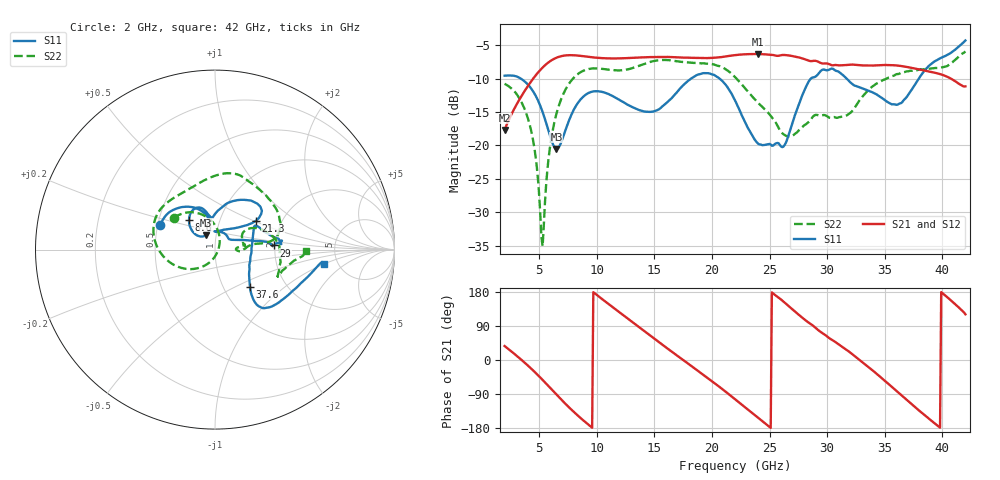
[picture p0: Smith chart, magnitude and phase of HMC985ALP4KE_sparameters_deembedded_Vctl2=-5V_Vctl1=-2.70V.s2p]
!s2p File: Measurements: S11, S21, S12, S22
# GHz S dB R 50.0
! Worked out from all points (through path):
!   401 points, 2 GHz to 42 GHz, reference 50 ohm
!   highest |S21| = -6.29 dB at 24 GHz (marker M1); lowest = -17.7 dB at 2 GHz (marker M2)
!   lowest |S11| = -20.5 dB at 6.5 GHz (marker M3), VSWR 1.21, Z = 44.8 + j7.26 ohm
!   |S11| at or under -10 dB: 3.42 GHz to 18.17 GHz (14.76 GHz wide, 137 % of centre); 20.67 GHz to 28.58 GHz (7.911 GHz wide, 32.1 % of centre); 31.7 GHz to 37.95 GHz (6.251 GHz wide, 18 % of centre)
!   |S22| runs from -35.1 to -5.9 dB; largest |S21 - S12| = 0.00063
!   S11 on the Smith chart (normalised r, x): 2 GHz: 0.52, +0.16; 8.6 GHz: 0.71, +0.25; 21.3 GHz: 1.48, +0.51; 29 GHz: 1.97, +0.10; 37.6 GHz: 1.33, -0.60; 42 GHz: 3.87, -1.01
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2  -9.55 156.1  -17.66 36.9  -17.67 36.9  -10.76 142.4
4.1  -11.02 121.8  -10.90 -16.8  -10.90 -16.8  -16.40 94.2
4.6  -12.25 112.5  -9.71 -31.2  -9.71 -31.2  -20.55 77.2
5.3  -14.99 101.8  -8.32 -52.6  -8.33 -52.6  -35.09 -32.9
5.9  -18.30 101.7  -7.44 -71.8  -7.44 -71.8  -20.76 -118.1
6.5  -20.55 121.2  -6.86 -91.1  -6.86 -91.1  -15.24 -141.0
8.6  -13.09 130.8  -6.58 -153.2  -6.58 -153.2  -9.02 165.3
8.7  -12.91 129.6  -6.60 -155.8  -6.61 -155.8  -8.92 163.4
12.4  -13.60 102.2  -6.93 116.1  -6.93 116.1  -8.69 113.1
15.4  -14.58 92.5  -6.75 47.2  -6.76 47.2  -7.24 77.8
18.2  -9.97 61.0  -6.86 -15.6  -6.87 -15.6  -7.60 54.3
21.3  -11.15 35.2  -6.63 -86.3  -6.64 -86.3  -8.71 14.5
22  -13.22 38.1  -6.46 -103.4  -6.47 -103.4  -9.74 9.3
24  -19.73 81.7  -6.29 -152.2  -6.30 -152.2  -13.60 8.0
26.3  -19.95 34.1  -6.45 151.5  -6.45 151.5  -18.43 -1.4
28.7  -9.84 3.9  -7.35 92.3  -7.36 92.3  -15.83 8.8
29  -9.67 4.0  -7.33 84.7  -7.33 84.7  -15.42 7.1
32.4  -11.05 23.9  -7.91 10.1  -7.91 10.1  -14.32 32.2
35.4  -13.63 7.3  -7.95 -65.2  -7.95 -65.1  -9.80 14.4
37.6  -10.95 -46.7  -8.46 -123.5  -8.46 -123.5  -8.71 -5.0
39.6  -7.15 -47.2  -9.21 -173.6  -9.21 -173.6  -8.41 -23.1
42  -4.27 -7.7  -11.15 120.5  -11.15 120.6  -5.90 -0.8
